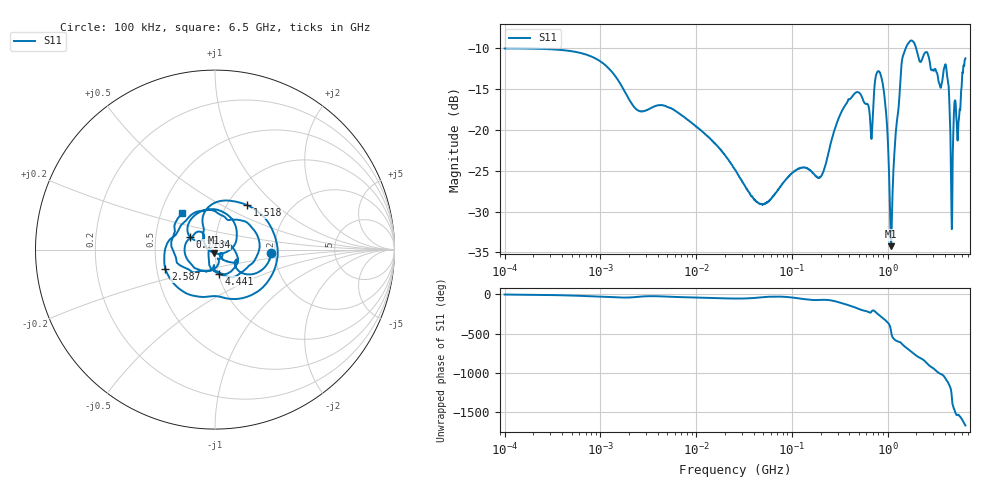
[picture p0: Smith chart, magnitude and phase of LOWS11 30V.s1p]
!Keysight Technologies,E5080B,MY59100498,A.17.05.10
!Date: Wednesday, August 30, 2023 18:49:10
!Correction: S11(C  1-Port  )
!S1P File: Measurement: S11:Log Frequency Sweep
# Hz S  dB  R 50
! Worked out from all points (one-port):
!   1601 points, 100 kHz to 6.5 GHz, reference 50 ohm
!   lowest |S11| = -34.2 dB at 1.089 GHz (marker M1), VSWR 1.04, Z = 49.2 - j1.76 ohm
!   |S11| at or under -10 dB: start of sweep to 1.554 GHz; 1.981 GHz to end of sweep
!   S11 on the Smith chart (normalised r, x): 100 kHz: 1.91, -0.07; 718.4 MHz: 0.75, +0.11; 1.518 GHz: 1.23, +0.67; 2.587 GHz: 0.56, -0.13; 4.441 GHz: 1.00, -0.27; 6.5 GHz: 0.64, +0.28
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100000  -10.08 -3.2
399589.6  -10.27 -12.7
1596718  -14.30 -41.4
2487396  -17.67 -32.0
6380321  -17.88 -34.5
2.54951e7  -24.89 -54.0
4.888947e7  -29.17 -37.9
1.018758e8  -25.26 -41.9
2.008454e8  -25.74 -70.9
4.070849e8  -16.24 -146.6
6.702952e8  -20.52 129.6
7.183677e8  -15.99 152.8
7.860529e8  -12.92 111.9
8.904243e8  -14.38 58.6
9.675956e8  -18.09 20.5
1.088507e9  -34.23 -113.2
1.330654e9  -15.90 115.4
1.517814e9  -10.30 54.2
1.626669e9  -9.54 25.9
2.002356e9  -10.19 -61.2
2.587259e9  -10.54 -158.4
3.274269e9  -13.03 97.7
4.115103e9  -12.64 -10.8
4.440884e9  -17.36 -81.7
4.759378e9  -26.54 47.7
5.065506e9  -16.41 -53.7
5.777982e9  -16.99 -122.7
6.5e9  -11.29 132.0
